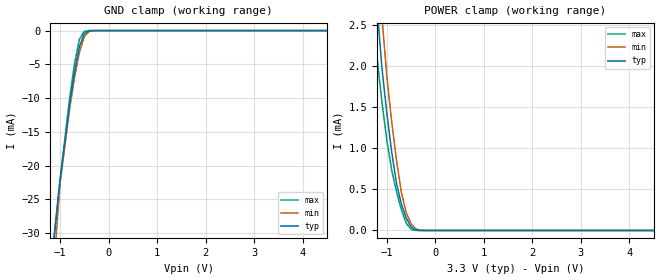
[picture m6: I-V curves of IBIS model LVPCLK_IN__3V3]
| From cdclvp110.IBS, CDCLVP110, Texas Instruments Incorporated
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|   Diff. Receiver Input Model for 3.3V VCC range   |
[Model]   LVPCLK_IN__3V3
Model_type   Input
| Signals   CLK0_T, CLK1_T,CLK0_N, CLK1_N
| variable   typ   min   max
C_comp   0.5pF   NA   NA
| Vicm(typ)=(VCC-0.3V-1V)=3.300V-1.3V=2.0V/2+1V ==>2.0V +/-0.25V
| Vicm(min)=(+1V) ==> 1.25V +/-0.25V
| Vicm(max)=(VCC-0.3V)=3.80V-0.3V ==> 3.50V +/-0.25V
Vinl = 1.75V   |
Vinh = 2.25V   |
[Model Spec]
|   VCC=3.3V   VCC=3.0V   VCC=3.8V
Vinl   1.75V   1.00V   3.25V
Vinh   2.25V   1.50V   3.75V
[Temperature Range]   40C   110C   -40C
[Voltage range]   3.3V   3.0V   3.8V
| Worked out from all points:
|   GND clamp passes 1 mA (typ) near -0.53 V on its own axis
|   POWER clamp passes 1 mA (typ) near -0.91 V on its own axis
[POWER Clamp]
|   40C:3.3V:nominal   110C:3.0V:weak   -40C:3.8:strong
|  Voltage   I(typ)   I(min)   I(max)
-3.9V     153.7mA    162.4mA    154.7mA
-1.3V     3.643mA    4.656mA    2.801mA
-1.2V     2.693mA    3.533mA    2.089mA
-1.1V     1.967mA    2.582mA    1.557mA
-1V       1.421mA    1.869mA    1.094mA
-900mV    952.2uA    1.32mA     732.8uA
-800mV    568.8uA    847.8uA    469uA
-700mV    320.1uA    460.6uA    250.5uA
-600mV    150.9uA    214.6uA    89.13uA
-500mV    43.24uA    80.19uA    12.52uA
-200mV    10.05nA    132.3nA    631.1pA
7.6V      -754.3pA   -13.44nA   -644.7pA
[GND Clamp]
|   40C:3.3V:nominal   110C:3.0V:weak   -40C:3.8:strong
|  Voltage   I(typ)   I(min)   I(max)
-3.8V     -426.9mA   -478.8mA   -379.4mA
-1.2V     -36.15mA   -42.21mA   -35.95mA
-1V       -22.25mA   -22.78mA   -22.21mA
-800mV    -10.9mA    -11.56mA   -9.953mA
-700mV    -6.1mA     -6.953mA   -4.88mA
-600mV    -2.375mA   -3.219mA   -1.316mA
-500mV    -439.4uA   -906.1uA   -101.6uA
-400mV    -35.43uA   -131.9uA   -2.723uA
-200mV    -62.78nA   -869.6nA   -560.2pA
7.6V      1.072nA    18.52nA    1.398nA
